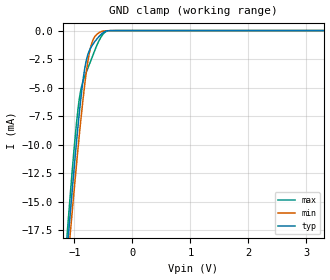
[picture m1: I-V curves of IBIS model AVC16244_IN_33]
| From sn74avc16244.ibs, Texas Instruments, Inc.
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[Model]   AVC16244_IN_33
Model_type  Input
Vinl=0.8
Vinh=2.0
| variable   typ   min   max
C_comp   4.57pF   3.04pF   8.95pF
[Temperature Range]   40   100   -40
| Ambient temperature   25   85   -40
[Voltage range]   3.3   3   3.6
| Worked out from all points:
|   GND clamp passes 1 mA (typ) near -0.65 V on its own axis
[GND Clamp]
| AVC16244_IN_33
|   Voltage   I(typ)   I(min)   I(max)
-3.3V     -168.5mA   -163mA     -178.3mA
-1.12V    -19.03mA   -20.7mA    -17.59mA
-1.1V     -17.8mA    -19.52mA   -16.29mA
-1.065V   -15.67mA   -17.48mA   -14.04mA
-985mV    -10.99mA   -12.94mA   -9.268mA
-930mV    -8.006mA   -9.963mA   -6.584mA
-885mV    -5.803mA   -7.664mA   -5.121mA
-825mV    -3.453mA   -4.886mA   -4.059mA
-715mV    -1.486mA   -1.371mA   -2.62mA
-570mV    -491.5uA   -175.5uA   -837.3uA
-370mV    -4.241uA   -4.164uA   -3.93uA
3.3V      220.5pA    727.1pA    16.58pA
